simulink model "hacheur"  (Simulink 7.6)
settings: Solver=ode23tb  StartTime=0.0  StopTime=10  RelTol=1e-3
StopFcn:
  | load UR_IR_hacheur.mat
  | plot(z(1,:),z(2,:),z(1,:),z(3,:))
  | axis([0 10 -1 15])
  | grid
  | title('hacheur - tension et courant dans la charge R')
  | xlabel('temps')
libraries: powerlib x10

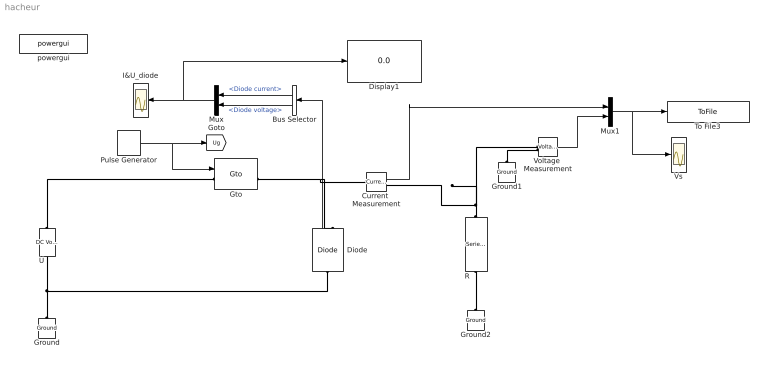
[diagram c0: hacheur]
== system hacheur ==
  Bus Selector : BusSelector  OutputSignals=Diode current,Diode voltage
  Current  Measurement : powerlib/Measurements/Current Measurement  DialogController=POWERSYS.PowerSysDialog  SystemSampleTime=-1  PhasorSimulation=off  OutputType=Complex  PSBequivalent=0
  Diode : powerlib/Power Electronics/Diode  DialogController=POWERSYS.PowerSysDialog  SystemSampleTime=-1  Ron=0.001  Lon=0  Vf=0.8  IC=0  UseSnubber=off  Rs=500  Cs=250e-9  Measurements=on
  Display1 : Display
  Ground : powerlib/Elements/Ground  DialogController=POWERSYS.PowerSysDialog  PhysicalDomain=powersysdomain  SubClassName=unknown  LeftPortType=p1  RightPortType=p1  LConnTagsString=a
  Ground1 : powerlib/Elements/Ground  DialogController=POWERSYS.PowerSysDialog  PhysicalDomain=powersysdomain  SubClassName=unknown  LeftPortType=p1  RightPortType=p1  LConnTagsString=a
  Ground2 : powerlib/Elements/Ground  DialogController=POWERSYS.PowerSysDialog  PhysicalDomain=powersysdomain  SubClassName=unknown  LeftPortType=p1  RightPortType=p1  LConnTagsString=a
  Gto : powerlib/Power Electronics/Gto  DialogController=POWERSYS.PowerSysDialog  SystemSampleTime=-1  Ron=0.001  Lon=0  Vf=1  Tf=10e-6  Tt=20e-6  IC=0  Rs=1e5  Cs=inf  Measurements=on
  I&U_diode : Scope
  Mux : Mux  Inputs=2
  Mux1 : Mux  Inputs=2
  Pulse Generator : DiscretePulseGenerator  PulseType=Time based  PulseWidth=60
  R : powerlib/Elements/Series RLC Branch  DialogController=POWERSYS.PowerSysDialog  PhysicalDomain=powersysdomain  SubClassName=unknown  LeftPortType=p1  RightPortType=p1  LConnTagsString=__new0  RConnTagsString=__new0  BranchType=R  Resistance=2  Inductance=1e-3  SetiL0=off  InitialCurrent=0  Capacitance=1e-6  Setx0=off  InitialVoltage=0  Measurements=None
  To File3 : ToFile  Filename=UR_IR_hacheur  MatrixName=z
  U : powerlib/Electrical Sources/DC Voltage Source  DialogController=POWERSYS.PowerSysDialog  SystemSampleTime=-1  Amplitude=15  Measurements=None
  Voltage  Measurement : powerlib/Measurements/Voltage Measurement  DialogController=POWERSYS.PowerSysDialog  SystemSampleTime=-1  PhasorSimulation=off  OutputType=Complex  PSBequivalent=0
  Vs : Scope
  powergui : powerlib/powergui  Priority=2  SystemSampleTime=-1  SimulationMode=Continuous  SampleTime=0  frequency=60  SPID=off  DisableSnubberDevices=off  DisableRonSwitches=off  DisableVfSwitches=off  SwTol=0  Interpol=off  frequencyindice=0  echomessages=off  HookPort=off  DisplayEquations=off  FunctionMessages=off  EnableUseOfTLC=off  x0status=blocks  RestoreLinks=warning  ResistiveCurrentMeasurement=off  Frange=logspace(0,3,50)  Ylog=off  Xlog=off  ShowGrid=off  save=off  variable=ZData  ZoomFFT=on  StartTime=0.0  cycles=1  DisplayStyle=off  fundamental=60  FreqAxis=off  MaxFrequency=1000  frequencyindicesteady=1  RmsSteady=1  display=off  Ts=0  methode=off
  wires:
  Pulse Generator/1 -> Gto/1, [Ug]
  Voltage  Measurement/1 -> Mux1/2
  Diode/1 -> Bus Selector/1
  Bus Selector/1 -> Mux/1  "<Diode current>"
  Bus Selector/2 -> Mux/2  "<Diode voltage>"
  Mux/1 -> I&U_diode/1, Display1/1
  Current  Measurement/1 -> Mux1/1
  Mux1/1 -> To File3/1, Vs/1
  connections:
  Diode/LConn1 -- U/LConn1 -- Ground/LConn1
  U/RConn1 -- Gto/LConn1
  Gto/RConn1 -- Diode/RConn1 -- Current  Measurement/LConn1
  Ground1/LConn1 -- Voltage  Measurement/LConn2
  R/RConn1 -- Ground2/LConn1
  R/LConn1 -- Current  Measurement/RConn1 -- Voltage  Measurement/LConn1
